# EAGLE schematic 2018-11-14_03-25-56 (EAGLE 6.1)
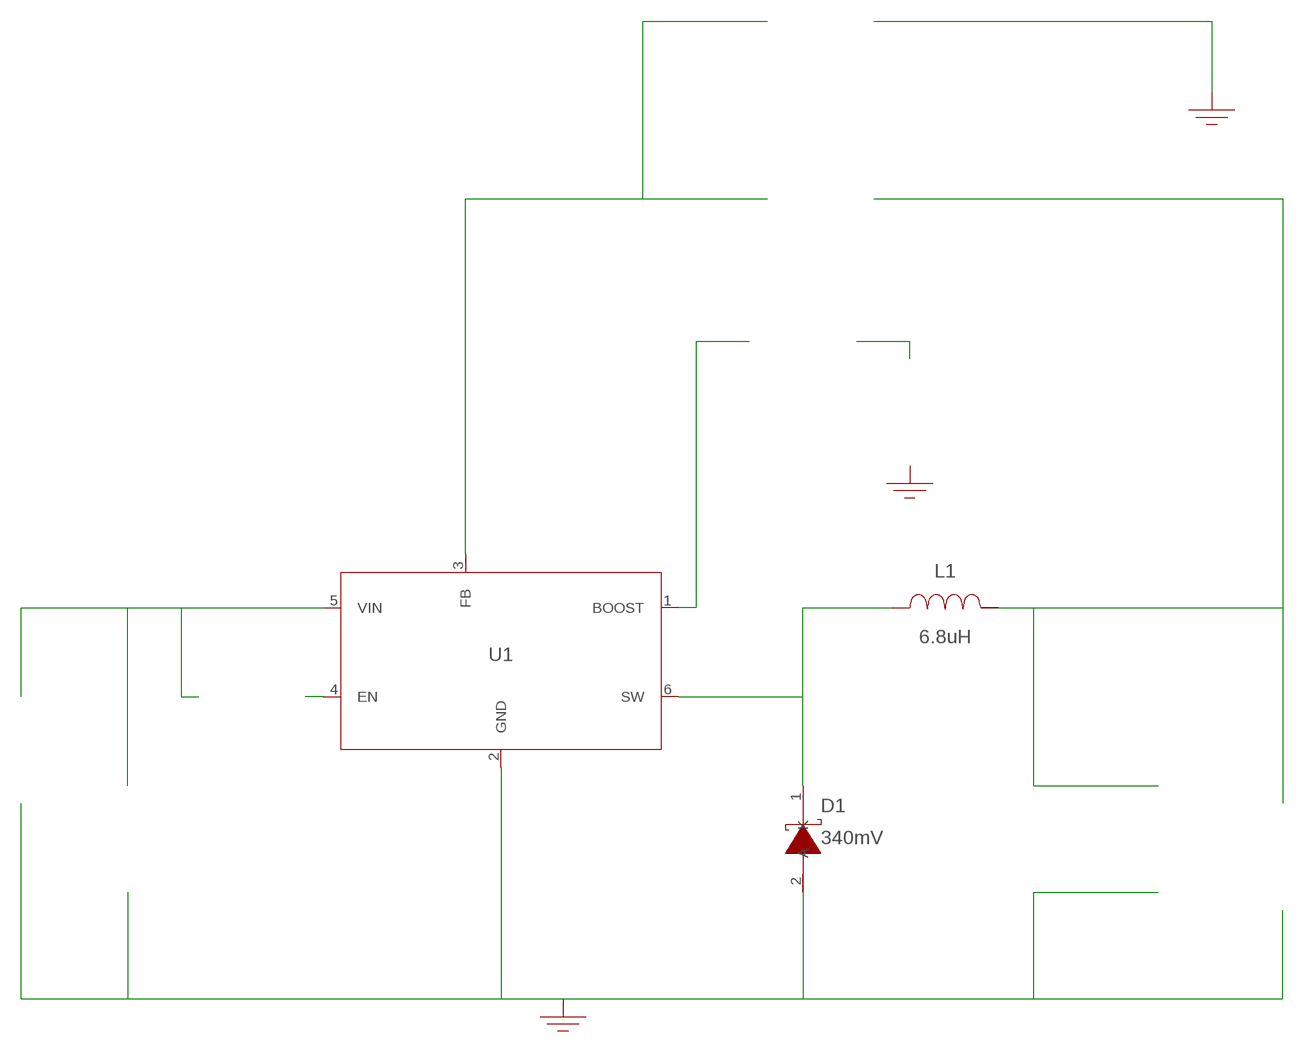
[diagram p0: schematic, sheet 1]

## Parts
CB  10nF  CGA4C2C0G1H103J060AACGA4C2C0G1H103J060AA  [0805]  (not placed on a sheet)
CIN  22uF  C2012X5R1V226M125ACC2012X5R1V226M125AC  [0805]  (not placed on a sheet)
COUT  10uF  C0805C106K8PACTUC0805C106K8PACTU  [0805]  (not placed on a sheet)
COUT_2  10uF  C0805C106K8PACTUC0805C106K8PACTU  [0805]  (not placed on a sheet)
D1  340mV  MBR1020VLMBR1020VL  [SOD-123F]
DBOOST  550mV  SS14FLSS14FL  [SOD-123F]  (not placed on a sheet)
GND  WB_GND  WB_GNDWB_GND  [WB_GND]
GND2  WB_GND  WB_GNDWB_GND  [WB_GND]
GND_12  WB_GND  WB_GNDWB_GND  [WB_GND]
IOUT  WB_CURRENT_LOAD  WB_CURRENT_LOADWB_CURRENT_LOAD  [WB_CURRENT_LOAD]  (not placed on a sheet)
L1  6.8uH  SRN3015-6R8MSRN3015-6R8M  [SRN3015]
RENABLE  10k  RC0201FR-0710KLRC0201FR-0710KL  [0201]  (not placed on a sheet)
RFB1  10k  RC0201FR-0710KLRC0201FR-0710KL  [0201]  (not placed on a sheet)
RFB2  34k  CRCW040234K0FKEDCRCW040234K0FKED  [0402]  (not placed on a sheet)
U1  LM2736XMK/NOPB  LM2736XMK/NOPBLM2736XMK/NOPB  [MK06A]
VIN  WB_BATTERY  WB_BATTERYWB_BATTERY  [WB_BATTERY]  (not placed on a sheet)
VSUPPLY  WB_PRIMITIVE_BATTERY  WB_PRIMITIVE_BATTERYWB_PRIMITIVE_BATTERY  [WB_PRIMITIVE_BATTERY]  (not placed on a sheet)

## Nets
0: Cin.2@2 Cout.2@2 Cout_2.2@2 D1.2(A) GND2.1 GND.1 GND_12.1 Iout.-@2 Rfb1.2@2 U1.2(GND) Vin.-@2 Vsupply.-@2
1: Cin.1@1 Renable.2@2 U1.5(VIN) Vin.+@1
2: Cb.1@1 Dboost.K@2 U1.1(BOOST)
3: Dboost.A@1 Vsupply.+@1
4: Rfb1.1@1 Rfb2.2@2 U1.3(FB)
5: Cout.1@1 Cout_2.1@1 Iout.+@1 L1.2 Rfb2.1@1
6: Cb.2@2 D1.1(K) L1.1 U1.6(SW)
7: Renable.1@1 U1.4(EN)
Unconnected: CB.1 CB.2 CIN.1 CIN.2 COUT.1 COUT.2 COUT_2.1 COUT_2.2 DBOOST.1(K) DBOOST.2(A) IOUT.1(+) IOUT.2(-) RENABLE.1 RENABLE.2 RFB1.1 RFB1.2 RFB2.1 RFB2.2 VIN.1(+) VIN.2(-) VSUPPLY.1(+) VSUPPLY.2(-)

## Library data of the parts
CB = AcceleratedDesigns_Lib:CGA4C2C0G1H103J060AA; Cap: 1.0E-8; Datasheet_URL: http://product.tdk.com/capacitor/mlcc/en/documents/mlcc%5Fautomotive%5Fgeneral%5Fen.pdf; ESR: 0.0; IRMS: 0.0; Manufacturer_Name: TDK; Manufacturer_Part_Number: CGA4C2C0G1H103J060AA; VDC: 50.0; Vendor: TDK
CIN = AcceleratedDesigns_Lib:C2012X5R1V226M125AC; Cap: 2.2E-5; Datasheet_URL: https://product.tdk.com/en/search/capacitor/ceramic/mlcc/info?part%5Fno%3DC2012X5R1V226M125AC; ESR: 0.00205; IRMS: 4.55587; Manufacturer_Name: TDK; Manufacturer_Part_Number: C2012X5R1V226M125AC; VDC: 35.0; Vendor: TDK
COUT COUT_2 = AcceleratedDesigns_Lib:C0805C106K8PACTU; Cap: 1.0E-5; ESR: 0.0030; IRMS: 11.43; Manufacturer_Name: Kemet; Manufacturer_Part_Number: C0805C106K8PACTU; VDC: 10.0; Vendor: Kemet
D1 = AcceleratedDesigns_Lib:MBR1020VL; Datasheet_URL: https://www.fairchildsemi.com/datasheets/MB/MBR1020VL.pdf; Io: 1.0; Manufacturer_Name: Fairchild Semiconductor; Manufacturer_Part_Number: MBR1020VL; VFatIo: 0.34; VRRM: 20.0; Vendor: Fairchild Semiconductor
DBOOST = AcceleratedDesigns_Lib:SS14FL; Datasheet_URL: https://www.fairchildsemi.com/datasheets/SS/SS13FL.pdf; Io: 1.0; Manufacturer_Name: Fairchild Semiconductor; Manufacturer_Part_Number: SS14FL; VFatIo: 0.55; VRRM: 40.0; Vendor: Fairchild Semiconductor
GND GND2 GND_12 = AcceleratedDesigns_Lib:WB_GND; Manufacturer_Name: WB_GND; Manufacturer_Part_Number: WB_GND; PowerPortType: POWER_GROUND; Value: Value
IOUT = AcceleratedDesigns_Lib:WB_CURRENT_LOAD; Manufacturer_Name: WB_CURRENT_LOAD; Manufacturer_Part_Number: WB_CURRENT_LOAD; PowerPortType: POWER_GROUND; Value: Value
L1 = AcceleratedDesigns_Lib:SRN3015-6R8M; DCR: 0.211; Datasheet_URL: http://www.bourns.com/data/global/pdfs/SRN3015.pdf; IDC: 1.05; L: 6.8E-6; Manufacturer_Name: Bourns; Manufacturer_Part_Number: SRN3015-6R8M; Vendor: Bourns
RENABLE RFB1 = AcceleratedDesigns_Lib:RC0201FR-0710KL; Datasheet_URL: http://www.yageo.com/documents/recent/PYu%2DRC%5FGroup%5F51%5FRoHS%5FL%5F5.pdf; Manufacturer_Name: Yageo; Manufacturer_Part_Number: RC0201FR-0710KL; Power: 0.05; Resistance: 10000.0; Tolerance: 1.0; Vendor: Yageo America
RFB2 = AcceleratedDesigns_Lib:CRCW040234K0FKED; Manufacturer_Name: Vishay-Dale; Manufacturer_Part_Number: CRCW040234K0FKED; Power: 0.063; Resistance: 34000.0; Tolerance: 1.0; Vendor: Vishay-Dale
U1 = AcceleratedDesigns_Lib:LM2736XMK/NOPB; Datasheet_URL: http://www.ti.com/product/lm2736x; Frequency: 1600000.0; Imax: 0.75; Manufacturer_Name: Texas Instruments; Manufacturer_Part_Number: LM2736XMK/NOPB; Mktg_Package: NA; NSID: LM2736XMK/NOPB; Package: NA; Vendor: Texas Instruments
VIN = AcceleratedDesigns_Lib:WB_BATTERY; Manufacturer_Name: WB_BATTERY; Manufacturer_Part_Number: WB_BATTERY; PowerPortType: POWER_GROUND; Value: Value
VSUPPLY = AcceleratedDesigns_Lib:WB_PRIMITIVE_BATTERY; Manufacturer_Name: WB_PRIMITIVE_BATTERY; Manufacturer_Part_Number: WB_PRIMITIVE_BATTERY; PowerPortType: POWER_GROUND; Value: Value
